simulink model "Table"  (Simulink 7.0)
settings: Solver=FixedStepDiscrete  SolverMode=SingleTasking  StartTime=0.0  StopTime=inf  FixedStep=samplePeriod  RelTol=1e-3  AbsTol=1e-6
PreLoadFcn:
  | initialize
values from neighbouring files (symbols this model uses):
  acal = acal(:)    [initialize.m]
  actParams = [	bulkModulus   * pressCanon    [initialize.m]
  atype = []    [displA2T.m]    (also in displEnvelope.m = varargin{1}{6}; displJacobian.m = ones(nact, 1); displT2A.m; forceA2T.m)
  dcal = dcal(:)    [initialize.m]
  fcal = fcal(:)    [initialize.m]
  forceCanon = 0.00444822    [initialize.m]
  inertia = inertia + inertiaP2Q([0 0 0], massA(i), cgA(:,i)-cg,  									inertiaCanon, massCanon)    [initialize.m]
  inertiaMask = zeros(3, 1)    [initialize.m]
  lengthCanon = 25.4    [initialize.m]
  mass = ones(3, 1) * (sum(massA) + massT + massS)    [initialize.m]
  massMask = zeros(3, 1)    [initialize.m]
  nUDPInp = nAct+nAcc+nAct    [initialize.m]
  nUDPOut = nAct    [initialize.m]
  returnPress = 50    [initialize.m]
  rtg = cg    [initialize.m]
  samplePeriod = controlPeriod/upsampleFactor    (= 0.00048828125)    [initialize.m]    (also in viewer.m = eval(getHeaderValue(header, 'DELTA_T')))
  staticForce = forceT2A(ftbl, dtbl0, dof, rh, rb, rl, canon, atype)    [initialize.m]
  upsampleFactor = 2    [initialize.m]
undefined symbols (not defined in the file or in its folder): animation, friction, yieldDispl
libraries: LibTransforms x9, LibDynamics x6

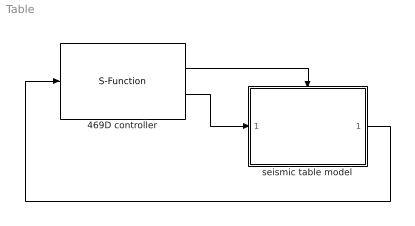
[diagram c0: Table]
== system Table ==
  469D controller : S-Function  FunctionName=ConnectUdpSimulink  Parameters=5002,nUDPInp,nUDPOut,upsampleFactor
  seismic table model : Subsystem  TreatAsAtomicUnit=on
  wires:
  469D controller/2 -> seismic table model/1(inp)
  469D controller/1 -> seismic table model/Trigger
  seismic table model/1(out) -> 469D controller/1

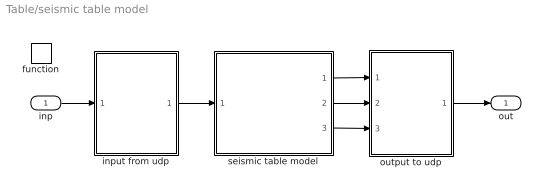
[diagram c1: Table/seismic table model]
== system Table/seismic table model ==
  inp : Inport  OutDataType=sfix(16)  OutScaling=2^0
  function : TriggerPort  TriggerType=function-call
  input from udp : Subsystem
  output to udp : Subsystem
  seismic table model : Subsystem
  out : Outport  OutDataType=sfix(16)  OutScaling=2^0
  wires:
  input from udp/1(valve cmd) -> seismic table model/1(valve cmd)
  inp/1 -> input from udp/1(inp)
  output to udp/1(out) -> out/1
  seismic table model/1(displ) -> output to udp/1(displ fbk)
  seismic table model/2(accel) -> output to udp/2(accel fbks)
  seismic table model/3(force) -> output to udp/3(force fbk)

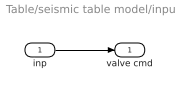
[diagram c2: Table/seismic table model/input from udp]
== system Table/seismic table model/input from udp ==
  inp : Inport  OutDataType=sfix(16)  OutScaling=2^0
  valve cmd : Outport  OutDataType=sfix(16)  OutScaling=2^0
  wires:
  inp/1 -> valve cmd/1

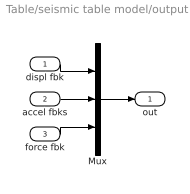
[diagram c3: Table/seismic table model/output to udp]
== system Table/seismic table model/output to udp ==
  displ fbk : Inport  OutDataType=sfix(16)  OutScaling=2^0
  accel fbks : Inport  Port=2  OutDataType=sfix(16)  OutScaling=2^0
  force fbk : Inport  Port=3  OutDataType=sfix(16)  OutScaling=2^0
  Mux : Mux  Inputs=3
  out : Outport  OutDataType=sfix(16)  OutScaling=2^0
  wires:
  force fbk/1 -> Mux/3
  accel fbks/1 -> Mux/2
  Mux/1 -> out/1
  displ fbk/1 -> Mux/1

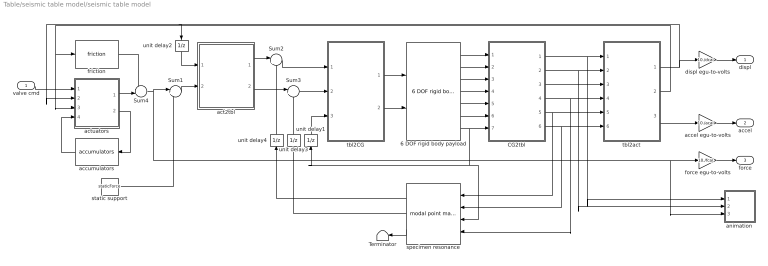
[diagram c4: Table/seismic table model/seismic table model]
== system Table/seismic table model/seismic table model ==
  valve cmd : Inport  OutDataType=sfix(16)  OutScaling=2^0
  6 DOF rigid body payload : LibDynamics/6 DOF rigid body payload  SystemSampleTime=-1  mass=mass.*massMask  inertia=diag(inertia.*inertiaMask)  gee=gee  massCanon=massCanon  inertiaCanon=inertiaCanon  linVelocCanon=linVelocCanon  linAccelCanon=linAccelCanon  rotDisplCanon=rotDisplCanon  rotVelocCanon=rotVelocCanon  rotAccelCanon=rotAccelCanon  rotForceCanon=rotForceCanon  initialPosition=zeros(6,1)  samplePeriod=samplePeriod
  CG2tbl : Subsystem  mask{ofst=-rtg}
      mask prompts: ofst "Origin offset"
  Sum1 : Sum  Inputs=|++  OutDataType=sfix(16)  OutScaling=2^0
  Sum2 : Sum  Inputs=|+-  OutDataType=sfix(16)  OutScaling=2^0
  Sum3 : Sum  Inputs=|+-  OutDataType=sfix(16)  OutScaling=2^0
  Sum4 : Sum  Inputs=-+|  OutDataType=sfix(16)  OutScaling=2^0
  Terminator : Terminator
  accel egu-to-volts : Gain  Gain=10./acal  ParameterDataType=sfix(16)  ParameterScaling=2^0  OutDataType=sfix(16)  OutScaling=2^0
  accumulators : LibDynamics/accumulators  Orientation=left  SystemSampleTime=-1  pumpFlow=pumpFlow  supplyPressure=supplyPress  precharge=precharge  bottleVolume=volume  gasConstant=gasConstant  flowCanon=flowCanon  volumeCanon=volumeCanon  samplePeriod=samplePeriod
  act2tbl : Subsystem
  actuators : Subsystem
  animation : Subsystem  mask{azim=-37.5, elev=35, params=animation, decim=ceil((1/samplePeriod)/32), samplePeriod=-1}
      mask prompts: azim "View azimuth (degrees)"; elev "View elevation (degrees)"; params "Parameters"; decim "Decimation factor"; samplePeriod "Sample period (sec)"
  displ egu-to-volts : Gain  Gain=10./dcal  ParameterDataType=sfix(16)  ParameterScaling=2^0  OutDataType=sfix(16)  OutScaling=2^0
  force egu-to-volts : Gain  Gain=10./fcal  ParameterDataType=sfix(16)  ParameterScaling=2^0  OutDataType=sfix(16)  OutScaling=2^0
  friction : LibDynamics/friction  SystemSampleTime=-1  friction=friction * forceCanon  yieldDispl=yieldDispl * lengthCanon  hysteresis=0  velocCanon=linVelocCanon  samplePeriod=samplePeriod
  specimen resonance : LibDynamics/modal point mass  Orientation=left  SystemSampleTime=-1  mass=modalMass  freq=modalFreq  damp=modalDamp  ofst=modalCG  gee=gee  massCanon=massCanon  linAccelCanon=linAccelCanon  rotDisplCanon=rotDisplCanon  rotVelocCanon=rotVelocCanon  rotForceCanon=rotForceCanon  samplePeriod=samplePeriod
  static support : Constant  Value=staticForce  OutDataType=sfix(16)  OutScaling=2^0
  tbl2CG : Subsystem  mask{ofst=rtg}
      mask prompts: ofst "Origin offset"
  tbl2act : Subsystem
  unit delay1 : UnitDelay  Orientation=up  X0=eye(3)  SampleTime=-1
  unit delay2 : UnitDelay  Orientation=down  SampleTime=-1
  unit delay3 : UnitDelay  Orientation=up  SampleTime=-1
  unit delay4 : UnitDelay  Orientation=up  SampleTime=-1
  displ : Outport  OutDataType=sfix(16)  OutScaling=2^0
  accel : Outport  Port=2  OutDataType=sfix(16)  OutScaling=2^0
  force : Outport  Port=3  OutDataType=sfix(16)  OutScaling=2^0
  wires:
  Sum4/1 -> animation/3(Fact), force egu-to-volts/1, Sum1/1
  actuators/1(force) -> Sum4/2
  friction/1 -> Sum4/1
  specimen resonance/2 -> unit delay3/1
  specimen resonance/1 -> unit delay4/1
  Sum3/1 -> tbl2CG/2(Frpw)
  act2tbl/2(Frpw) -> Sum3/1
  Sum2/1 -> tbl2CG/1(Fxyz)
  act2tbl/1(Fxyz) -> Sum2/1
  unit delay4/1 -> Sum2/2
  unit delay3/1 -> Sum3/2
  CG2tbl/6(Arpw) -> tbl2act/6(Arpw), specimen resonance/2
  CG2tbl/5(Axyz) -> tbl2act/5(Axyz), specimen resonance/1
  CG2tbl/4(Vrpw) -> tbl2act/4(Vrpw), specimen resonance/4
  CG2tbl/3(Vxyz) -> tbl2act/3(Vxyz)
  CG2tbl/2(rpw) -> animation/2(rpw), tbl2act/2(rpw)
  CG2tbl/1(xyz) -> animation/1(xyz), tbl2act/1(xyz)
  tbl2act/2(veloc act) -> friction/1, actuators/3(veloc)
  unit delay2/1 -> act2tbl/1(displ act)
  unit delay1/1 -> tbl2CG/3(DCM)
  tbl2act/3(accel act) -> accel egu-to-volts/1
  6 DOF rigid body payload/7 -> specimen resonance/3, unit delay1/1, CG2tbl/7(DCM)
  6 DOF rigid body payload/6 -> CG2tbl/6(accel rpw)
  6 DOF rigid body payload/5 -> CG2tbl/5(accel xyz)
  6 DOF rigid body payload/4 -> CG2tbl/4(veloc rpw)
  6 DOF rigid body payload/3 -> CG2tbl/3(veloc xyz)
  6 DOF rigid body payload/2 -> CG2tbl/2(displ rpw)
  6 DOF rigid body payload/1 -> CG2tbl/1(displ xyz)
  tbl2CG/1(force xyz) -> 6 DOF rigid body payload/1
  valve cmd/1 -> actuators/1(cmds)
  tbl2act/1(displ act) -> displ egu-to-volts/1, actuators/2(displ), unit delay2/1
  tbl2CG/2(force rpw) -> 6 DOF rigid body payload/2
  actuators/2(flow) -> accumulators/1
  accumulators/1 -> actuators/4(press)
  force egu-to-volts/1 -> force/1
  displ egu-to-volts/1 -> displ/1
  accel egu-to-volts/1 -> accel/1
  Sum1/1 -> act2tbl/2(force act)
  static support/1 -> Sum1/2
  specimen resonance/3 -> Terminator/1

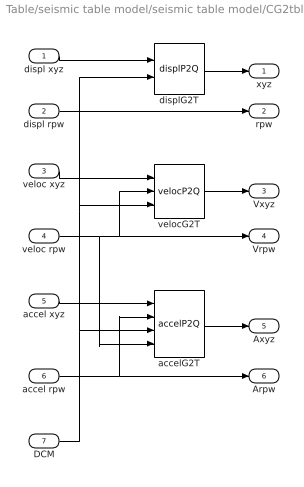
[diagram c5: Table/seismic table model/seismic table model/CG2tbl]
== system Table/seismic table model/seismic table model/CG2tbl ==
  displ xyz : Inport  OutDataType=sfix(16)  OutScaling=2^0
  displ rpw : Inport  Port=2  OutDataType=sfix(16)  OutScaling=2^0
  veloc xyz : Inport  Port=3  OutDataType=sfix(16)  OutScaling=2^0
  veloc rpw : Inport  Port=4  OutDataType=sfix(16)  OutScaling=2^0
  accel xyz : Inport  Port=5  OutDataType=sfix(16)  OutScaling=2^0
  accel rpw : Inport  Port=6  OutDataType=sfix(16)  OutScaling=2^0
  DCM : Inport  Port=7  OutDataType=sfix(16)  OutScaling=2^0
  accelG2T : LibTransforms/accelP2Q  SystemSampleTime=-1  dof=1:6  ofst=ofst
  displG2T : LibTransforms/displP2Q  SystemSampleTime=-1  dof=1:6  ofst=ofst
  velocG2T : LibTransforms/velocP2Q  SystemSampleTime=-1  dof=1:6  ofst=ofst
  xyz : Outport  OutDataType=sfix(16)  OutScaling=2^0
  rpw : Outport  Port=2  OutDataType=sfix(16)  OutScaling=2^0
  Vxyz : Outport  Port=3  OutDataType=sfix(16)  OutScaling=2^0
  Vrpw : Outport  Port=4  OutDataType=sfix(16)  OutScaling=2^0
  Axyz : Outport  Port=5  OutDataType=sfix(16)  OutScaling=2^0
  Arpw : Outport  Port=6  OutDataType=sfix(16)  OutScaling=2^0
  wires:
  accel rpw/1 -> accelG2T/2, Arpw/1
  DCM/1 -> accelG2T/3, velocG2T/3, displG2T/2
  veloc rpw/1 -> accelG2T/4, velocG2T/2, Vrpw/1
  veloc xyz/1 -> velocG2T/1
  accel xyz/1 -> accelG2T/1
  displ xyz/1 -> displG2T/1
  displG2T/1 -> xyz/1
  displ rpw/1 -> rpw/1
  velocG2T/1 -> Vxyz/1
  accelG2T/1 -> Axyz/1

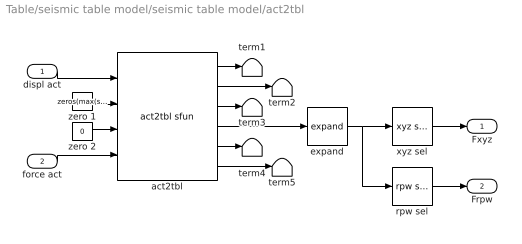
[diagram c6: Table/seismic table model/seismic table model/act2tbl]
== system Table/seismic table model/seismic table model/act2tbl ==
  displ act : Inport  OutDataType=sfix(16)  OutScaling=2^0
  force act : Inport  Port=2  OutDataType=sfix(16)  OutScaling=2^0
  act2tbl : LibTransforms/act2tbl sfun  atype=atype  nVel=0  nFrc=length(atype)  dof=dof  rh=rh  rb=rb  rl=rl  ra=[]  ea=[]  dmax=dmax  canon=canon  gee=gee  action=1  rate=0  count=1
  expand : LibTransforms/expand  SystemSampleTime=-1  size=6  elements=dof
  rpw sel : LibTransforms/rpw sel  SystemSampleTime=-1  dof=1:6
  term{1..5} (5 alike) : Terminator
  xyz sel : LibTransforms/xyz sel  SystemSampleTime=-1  dof=1:6
  zero 1 : Constant  Value=zeros(max(sum(dof>3), 1), 1)  OutDataType=sfix(16)  OutScaling=2^0
  zero 2 : Constant  Value=0  OutDataType=sfix(16)  OutScaling=2^0
  Fxyz : Outport  OutDataType=sfix(16)  OutScaling=2^0
  Frpw : Outport  Port=2  OutDataType=sfix(16)  OutScaling=2^0
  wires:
  rpw sel/1 -> Frpw/1
  force act/1 -> act2tbl/4
  xyz sel/1 -> Fxyz/1
  displ act/1 -> act2tbl/1
  act2tbl/4 -> expand/1
  zero 2/1 -> act2tbl/3
  zero 1/1 -> act2tbl/2
  act2tbl/1 -> term1/1
  act2tbl/2 -> term2/1
  act2tbl/3 -> term3/1
  act2tbl/5 -> term4/1
  act2tbl/6 -> term5/1
  expand/1 -> rpw sel/1, xyz sel/1

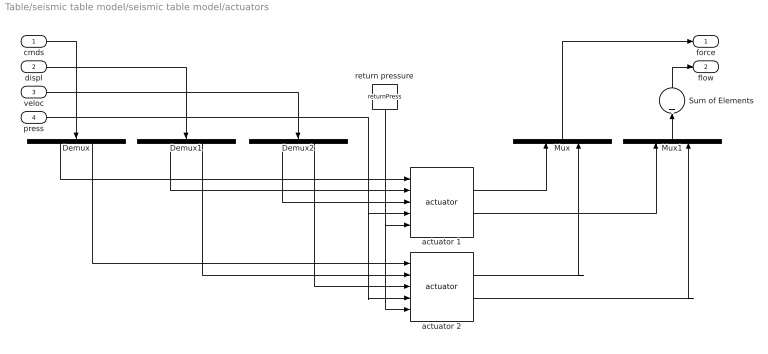
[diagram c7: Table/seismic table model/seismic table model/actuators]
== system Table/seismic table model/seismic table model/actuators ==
  cmds : Inport  OutDataType=sfix(16)  OutScaling=2^0
  displ : Inport  Port=2  OutDataType=sfix(16)  OutScaling=2^0
  veloc : Inport  Port=3  OutDataType=sfix(16)  OutScaling=2^0
  press : Inport  Port=4  OutDataType=sfix(16)  OutScaling=2^0
  Demux : Demux  Orientation=down  Outputs=nAct
  Demux1 : Demux  Orientation=down  Outputs=nAct
  Demux2 : Demux  Orientation=down  Outputs=nAct
  Mux : Mux  Orientation=up  Inputs=nAct
  Mux1 : Mux  Orientation=up  Inputs=nAct
  Sum of Elements : Sum  Orientation=up  Inputs=+  OutDataType=sfix(16)  OutScaling=2^-10
  actuator 1 : LibDynamics/actuator  SystemSampleTime=-1  params=actParams(:,1)
  actuator 2 : LibDynamics/actuator  SystemSampleTime=-1  params=actParams(:,2)
  return pressure : Constant  Orientation=down  Value=returnPress  OutDataType=sfix(16)  OutScaling=2^0
  force : Outport  OutDataType=sfix(16)  OutScaling=2^0
  flow : Outport  Port=2  OutDataType=sfix(16)  OutScaling=2^0
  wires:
  Mux/1 -> force/1
  cmds/1 -> Demux/1
  displ/1 -> Demux1/1
  Demux/1 -> actuator 1/1
  Demux/2 -> actuator 2/1
  Demux1/1 -> actuator 1/2
  Demux2/1 -> actuator 1/3
  Demux1/2 -> actuator 2/2
  Demux2/2 -> actuator 2/3
  actuator 1/1 -> Mux/1
  actuator 2/1 -> Mux/2
  veloc/1 -> Demux2/1
  press/1 -> actuator 1/4, actuator 2/4
  return pressure/1 -> actuator 1/5, actuator 2/5
  Mux1/1 -> Sum of Elements/1
  actuator 1/2 -> Mux1/1
  actuator 2/2 -> Mux1/2
  Sum of Elements/1 -> flow/1

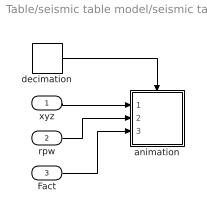
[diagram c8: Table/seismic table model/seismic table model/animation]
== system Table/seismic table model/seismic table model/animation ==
  xyz : Inport
  rpw : Inport  Port=2
  Fact : Inport  Port=3
  animation : Subsystem  TreatAsAtomicUnit=on
  decimation : DiscretePulseGenerator  Period=decim  SampleTime=samplePeriod
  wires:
  decimation/1 -> animation/Trigger
  xyz/1 -> animation/1(xyz)
  Fact/1 -> animation/3(Fact)
  rpw/1 -> animation/2(rpw)

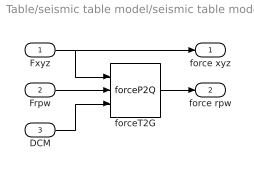
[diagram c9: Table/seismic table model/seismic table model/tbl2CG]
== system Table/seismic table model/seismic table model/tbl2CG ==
  Fxyz : Inport  OutDataType=sfix(16)  OutScaling=2^0
  Frpw : Inport  Port=2  OutDataType=sfix(16)  OutScaling=2^0
  DCM : Inport  Port=3  OutDataType=sfix(16)  OutScaling=2^0
  forceT2G : LibTransforms/forceP2Q  SystemSampleTime=-1  dof=1:6  ofst=ofst
  force xyz : Outport  OutDataType=sfix(16)  OutScaling=2^0
  force rpw : Outport  Port=2  OutDataType=sfix(16)  OutScaling=2^0
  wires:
  DCM/1 -> forceT2G/3
  forceT2G/1 -> force rpw/1
  Fxyz/1 -> force xyz/1, forceT2G/1
  Frpw/1 -> forceT2G/2

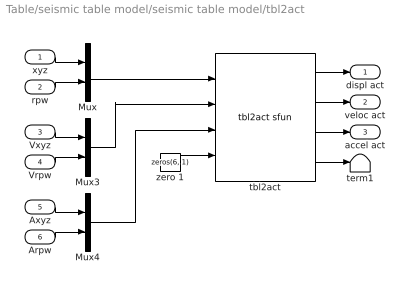
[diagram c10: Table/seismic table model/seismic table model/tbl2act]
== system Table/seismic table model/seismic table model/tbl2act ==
  xyz : Inport  OutDataType=sfix(16)  OutScaling=2^0
  rpw : Inport  Port=2  OutDataType=sfix(16)  OutScaling=2^0
  Vxyz : Inport  Port=3  OutDataType=sfix(16)  OutScaling=2^0
  Vrpw : Inport  Port=4  OutDataType=sfix(16)  OutScaling=2^0
  Axyz : Inport  Port=5  OutDataType=sfix(16)  OutScaling=2^0
  Arpw : Inport  Port=6  OutDataType=sfix(16)  OutScaling=2^0
  Mux : Mux  Inputs=2
  Mux3 : Mux  Inputs=2
  Mux4 : Mux  Inputs=2
  tbl2act : LibTransforms/tbl2act sfun  atype=atype  nVel=length(atype)  nFrc=0  dof=1:6  rh=rh  rb=rb  rl=rl  ra=ra  ea=ea  canon=canon  gee=gee  action=1  rate=0
  term1 : Terminator
  zero 1 : Constant  Value=zeros(6, 1)  OutDataType=sfix(16)  OutScaling=2^0
  displ act : Outport  OutDataType=sfix(16)  OutScaling=2^0
  veloc act : Outport  Port=2  OutDataType=sfix(16)  OutScaling=2^0
  accel act : Outport  Port=3  OutDataType=sfix(16)  OutScaling=2^0
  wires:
  tbl2act/1 -> displ act/1
  tbl2act/2 -> veloc act/1
  tbl2act/3 -> accel act/1
  tbl2act/4 -> term1/1
  zero 1/1 -> tbl2act/4
  xyz/1 -> Mux/1
  rpw/1 -> Mux/2
  Vxyz/1 -> Mux3/1
  Vrpw/1 -> Mux3/2
  Axyz/1 -> Mux4/1
  Arpw/1 -> Mux4/2
  Mux/1 -> tbl2act/1
  Mux3/1 -> tbl2act/2
  Mux4/1 -> tbl2act/3

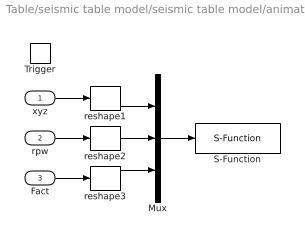
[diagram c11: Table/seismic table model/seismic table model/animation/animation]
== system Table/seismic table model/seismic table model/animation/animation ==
  xyz : Inport  OutDataType=sfix(16)  OutScaling=2^0
  rpw : Inport  Port=2  OutDataType=sfix(16)  OutScaling=2^0
  Fact : Inport  Port=3  OutDataType=sfix(16)  OutScaling=2^0
  Trigger : TriggerPort
  Mux : Mux  Inputs=3
  S-Function : S-Function  FunctionName=animation  Parameters=azim,elev,params
  reshape1 : Reshape
  reshape2 : Reshape
  reshape3 : Reshape
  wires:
  Mux/1 -> S-Function/1
  xyz/1 -> reshape1/1
  Fact/1 -> reshape3/1
  reshape3/1 -> Mux/3
  rpw/1 -> reshape2/1
  reshape2/1 -> Mux/2
  reshape1/1 -> Mux/1
